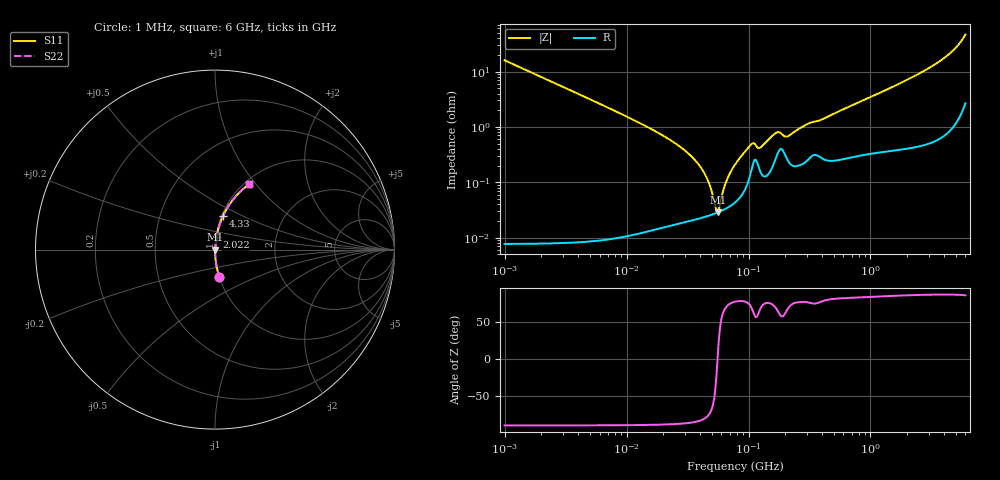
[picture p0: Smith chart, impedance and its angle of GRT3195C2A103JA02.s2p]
!Murata Part Number: GRT3195C2A103JA02
!These Parameters are Measured in Series Mode Connection
!Data Generated on Jun 19, 2026
!  o--ll--o
!Port1  Port2
!  o------o
!Operation Temp=25[degC], DC Bias Voltage=0[V]
!Freq. Start=1000[kHz] Stop=6[GHz] 401[Steps]
# Hz S RI R 50
!Freq.(Hz) S11(Real) S11(Imag) S21(Real) S21(Imag) S12(Real) S12(Imag) S22(Real) S22(Imag)
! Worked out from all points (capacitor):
!   401 points, 1 MHz to 6 GHz, reference 50 ohm
!   read as one part in series: C = 9.99 nF near 1.044 MHz
!   lowest |Z| = 28.7 mohm at 55.9 MHz (marker M1)
!   series resonance near 55.68 MHz, so ESL is about 820 pH
!   S11 on the Smith chart (normalised r, x): 1 MHz: 1.00, -0.32; 2.022 GHz: 1.01, +0.14; 4.33 GHz: 1.02, +0.40; 6 GHz: 1.05, +0.93
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1000000  0.0248 -0.1554  0.9752 0.1554  0.9752 0.1554  0.0248 -0.1554
4293785  0.00144 -0.0368  0.9986 0.0368  0.9986 0.0368  0.00144 -0.0368
1.843659e7  0.000204 -0.00767  0.9998 0.00767  0.9998 0.00767  0.000204 -0.00767
2.848316e7  0.000201 -0.00412  0.9998 0.00412  0.9998 0.00412  0.000201 -0.00412
3.8621e7  0.000223 -0.00214  0.9998 0.00214  0.9998 0.00214  0.000223 -0.00214
4.596069e7  0.000246 -0.00111  0.9998 0.00111  0.9998 0.00111  0.000246 -0.00111
4.905945e7  0.000257 -0.000733  0.9997 0.000733  0.9997 0.000733  0.000257 -0.000733
5.351853e7  0.000275 -0.00023  0.9997 0.00023  0.9997 0.00023  0.000275 -0.00023
5.589783e7  0.000286 2.28e-05  0.9997 -2.28e-05  0.9997 -2.28e-05  0.000286 2.28e-05
5.838291e7  0.000298 0.000277  0.9997 -0.000277  0.9997 -0.000277  0.000298 0.000277
6.23192e7  0.000318 0.000663  0.9997 -0.000663  0.9997 -0.000663  0.000318 0.000663
6.652088e7  0.000344 0.00106  0.9997 -0.00106  0.9997 -0.00106  0.000344 0.00106
7.745967e7  0.000435 0.00204  0.9996 -0.00204  0.9996 -0.00204  0.000435 0.00204
1.073387e8  0.00193 0.00462  0.9981 -0.00462  0.9981 -0.00462  0.00193 0.00462
1.249896e8  0.00156 0.00392  0.9984 -0.00392  0.9984 -0.00392  0.00156 0.00392
1.694764e8  0.00296 0.00728  0.997 -0.00728  0.997 -0.00728  0.00296 0.00728
2.106508e8  0.00249 0.00631  0.9975 -0.00631  0.9975 -0.00631  0.00249 0.00631
3.325952e8  0.00313 0.0117  0.9969 -0.0117  0.9969 -0.0117  0.00313 0.0117
1.428092e9  0.00605 0.049  0.994 -0.049  0.994 -0.049  0.00605 0.049
2.022471e9  0.0091 0.0708  0.9909 -0.0708  0.9909 -0.0708  0.0091 0.0708
4.329827e9  0.0452 0.1889  0.9548 -0.1889  0.9548 -0.1889  0.0452 0.1889
6e9  0.1921 0.3664  0.8079 -0.3664  0.8079 -0.3664  0.1921 0.3664
